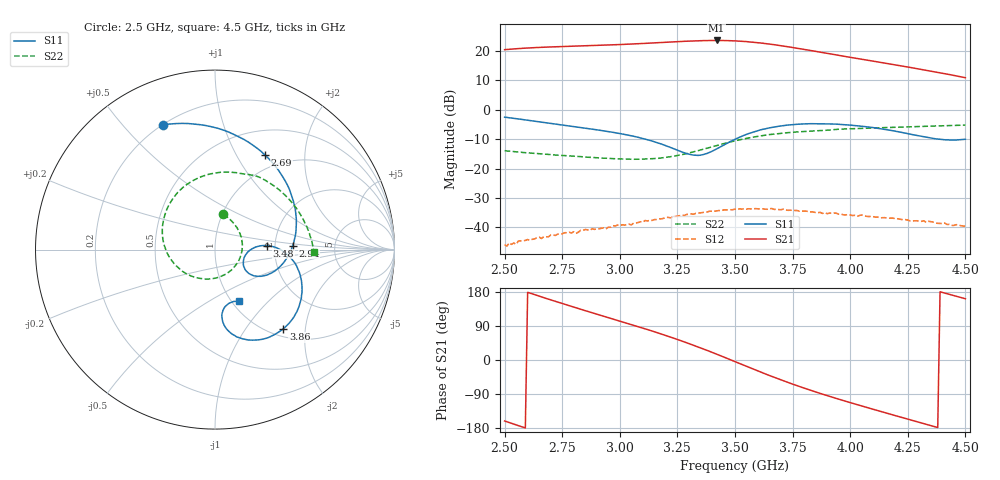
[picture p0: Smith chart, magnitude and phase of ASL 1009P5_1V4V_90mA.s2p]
!ASL 1009P5 : Low Noise Amplifier S-parameter data 2.5-4.5 GHz
!Bias conditions Vd1=1V, Vd2=4V, Total current=90 mA
!Date: Tuesday, January 09, 2007 14:24:47
!S2P File: Measurements: S11, S21, S12, S22:
# Hz S  dB  R 50
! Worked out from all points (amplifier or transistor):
!   201 points, 2.5 GHz to 4.5 GHz, reference 50 ohm
!   highest |S21| = 23.6 dB at 3.42 GHz (marker M1)
!   |S21| within 3 dB of that: 2.52 GHz to 3.796 GHz (1.276 GHz wide, 40.4 % of centre)
!   unconditionally stable (mu >= 1): start of sweep to end of sweep
!   at 2.83 GHz: K = 3.47, MAG = 23.0 dB, |S12| = -41.0 dB
!   at 3.5 GHz: K = 1.53, MAG = 24.3 dB, |S12| = -33.8 dB
!   at 4.5 GHz: K = 8.37, MAG = 13.0 dB, |S12| = -39.6 dB
!   S11 on the Smith chart (normalised r, x): 2.5 GHz: 0.20, +0.65; 2.69 GHz: 0.81, +1.32; 2.94 GHz: 2.52, +0.14; 3.48 GHz: 1.81, +0.09; 3.86 GHz: 1.14, -1.53; 4.5 GHz: 1.07, -0.69
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2.5e9  -2.47 112.5  20.48 -160.9  -45.85 120.9  -13.89 76.5
2.59e9  -3.40 88.7  21.01 -179.4  -44.40 99.9  -14.55 63.4
2.69e9  -4.50 62.2  21.37 160.6  -43.19 86.6  -15.14 47.5
2.84e9  -6.11 24.8  21.76 132.1  -41.00 58.3  -15.95 19.9
2.94e9  -7.26 2.9  22.01 113.8  -40.49 43.9  -16.44 -2.6
3.07e9  -9.15 -20.8  22.48 89.9  -38.49 20.8  -16.80 -38.6
3.17e9  -11.36 -33.0  22.88 70.7  -37.03 2.2  -16.45 -72.6
3.23e9  -13.10 -35.0  23.13 58.5  -36.37 -8.5  -15.79 -94.5
3.29e9  -14.87 -28.7  23.36 45.6  -35.56 -21.7  -14.86 -117.2
3.36e9  -15.24 -9.8  23.55 29.8  -34.91 -36.6  -13.43 -143.4
3.42e9  -13.29 2.5  23.61 15.5  -34.37 -50.5  -12.14 -165.0
3.48e9  -10.76 4.5  23.53 0.7  -33.97 -65.5  -10.88 174.5
3.5e9  -10.01 3.3  23.47 -4.3  -33.76 -71.0  -10.52 167.8
3.59e9  -7.28 -7.2  22.93 -26.7  -33.58 -91.7  -9.12 139.9
3.67e9  -5.81 -19.8  22.17 -45.9  -33.85 -110.2  -8.21 117.8
3.74e9  -5.10 -31.0  21.35 -61.5  -34.13 -124.9  -7.68 100.8
3.84e9  -4.70 -46.2  20.03 -82.3  -34.73 -146.6  -7.16 80.0
3.86e9  -4.69 -49.2  19.76 -86.3  -34.92 -149.4  -7.09 76.3
4e9  -5.18 -66.5  17.89 -112.4  -35.75 -175.6  -6.42 53.7
4.17e9  -6.89 -81.3  15.64 -142.3  -36.85 158.5  -5.98 31.6
4.33e9  -9.30 -82.7  13.49 -169.8  -38.28 129.1  -5.59 14.4
4.5e9  -9.99 -65.4  10.93 161.6  -39.61 104.2  -5.18 -1.5
